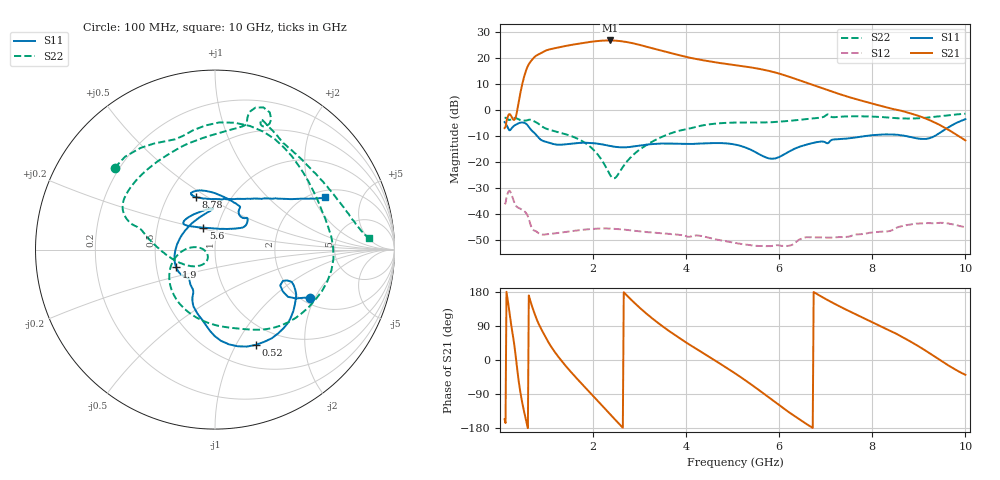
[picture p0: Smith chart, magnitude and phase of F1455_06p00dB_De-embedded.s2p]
! Integrated Device Technology
! Corporate Headquarters
! 6024 Silver Creek Valley Road
! San Jose, CA 95138  USA
! Phone:  1-408-284-8200
! Toll Free:  1-800-223-1366
! Webpage:  http://www.idt.com/
! Timing and RF Division
! 515 Groton Road, Suite 102
! Westford, MA 01886-6024
! Device:  F1455
! Description: 6-bit 0.5 dB Transmit Variable Gain Amplifier
! Frequency:  1400.0 -  2300.00 MHz
! Package:  6x6 mm Thin QFN Plastic Package: 28 pin
! State:  12
! Atten State:  6.0 dB
! Voltage:  +5.00 Volts
! Current:  217.708 mA
! Data:  The device was measured on a the F1455 evaluation board which has
!  individual transmission lines to the RF pins.  Data was collected
!  using a calibrated network analyzer.  The evaluation board was
!  de-embedded using a TRL calibration technique.
!  The reference plane is the edge of the package pin.
!  Pin  1 = CSb
!  Pin  2 = DATA
!  Pin  3 = CLK
!  Pin  4 = RSET
!  Pin  5 = GND
!  Pin  6 = RFIN  = Port 1
!  Pin  7 = GND
!  Pin  8 = NC
!  Pin  9 = NC
!  Pin 10 = NC
!  Pin 11 = NC
!  Pin 12 = NC
!  Pin 13 = NC
!  Pin 14 = /STBY
!  Pin 15 = GND
!  Pin 16 = RFOUT  = Port 2
!  Pin 17 = GND
!  Pin 18 = NC
!  Pin 19 = NC
!  Pin 20 = NC
!  Pin 21 = GND
!  Pin 22 = NC
!  Pin 23 = GND
!  Pin 24 = NC
!  Pin 25 = NC
!  Pin 26 = NC
!  Pin 27 = GND
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# GHz S dB R 50
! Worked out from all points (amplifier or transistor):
!   496 points, 100 MHz to 10 GHz, reference 50 ohm
!   highest |S21| = 26.9 dB at 2.36 GHz (marker M1)
!   |S21| within 3 dB of that: 1.173 GHz to 3.274 GHz (2.101 GHz wide, 94.5 % of centre)
!   unconditionally stable (mu >= 1): start of sweep to end of sweep
!   at 1.74 GHz: K = 4.52, MAG = 26.4 dB, |S12| = -46.0 dB
!   at 5.06 GHz: K = 15.06, MAG = 19.4 dB, |S12| = -51.0 dB
!   at 10 GHz: K = 46.17, MAG = -2.9 dB, |S12| = -45.0 dB
!   S11 on the Smith chart (normalised r, x): 100 MHz: 2.21, -1.84; 520 MHz: 0.76, -1.21; 1.9 GHz: 0.63, -0.13; 5.6 GHz: 0.85, +0.21; 8.78 GHz: 0.69, +0.44; 10 GHz: 2.30, +2.47
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0.1  -4.50 -26.8  -6.80 -156.7  -36.10 42.5  -2.84 140.8
0.4  -4.97 -41.1  2.88 -53.7  -37.48 -114.6  -3.43 50.4
0.52  -4.78 -66.9  12.99 -137.0  -38.76 -154.6  -3.96 23.7
0.7  -8.05 -100.6  19.69 137.8  -45.68 153.2  -3.88 -20.9
0.82  -10.29 -114.4  21.45 98.4  -47.11 138.4  -5.06 -49.5
0.96  -11.96 -119.4  22.78 64.8  -47.76 122.8  -6.78 -73.7
1.14  -12.91 -128.5  23.76 27.8  -47.38 99.3  -7.86 -98.1
1.34  -13.17 -133.5  24.52 -4.8  -46.92 77.0  -8.81 -121.8
1.76  -12.47 -149.1  25.86 -63.2  -45.94 40.7  -11.74 -160.5
1.9  -12.50 -156.5  26.24 -81.6  -45.73 30.3  -13.43 -171.2
2.12  -12.86 -171.8  26.70 -110.4  -45.47 14.9  -17.41 175.1
2.36  -13.66 165.2  26.89 -142.2  -45.45 -0.9  -24.62 -176.4
2.62  -14.23 135.4  26.57 -176.2  -45.77 -16.3  -22.32 -126.2
2.92  -13.75 107.3  25.55 147.2  -46.38 -31.2  -16.24 -143.0
3.4  -12.79 92.7  23.28 97.5  -47.20 -49.8  -10.87 -176.6
4.1  -12.92 113.6  20.16 38.4  -48.47 -72.1  -6.87 163.7
5.06  -13.18 140.6  17.38 -35.9  -51.01 -105.5  -4.69 148.3
5.6  -17.16 118.2  15.86 -82.5  -52.14 -112.7  -4.66 127.0
6.7  -12.65 40.0  9.91 -177.7  -48.77 -143.1  -3.13 78.4
8.36  -9.25 110.9  0.89 78.3  -46.47 165.3  -2.77 62.1
8.78  -10.13 110.3  -0.94 51.4  -44.03 150.7  -3.14 46.8
10  -3.39 25.4  -11.56 -39.0  -44.99 77.4  -1.29 4.5
